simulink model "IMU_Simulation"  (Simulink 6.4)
settings: Solver=FixedStepDiscrete  StartTime=0.0  StopTime=25  FixedStep=.001  RelTol=1e-3
PreLoadFcn:
  | Script_Kalman
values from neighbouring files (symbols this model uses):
  Az = [1 -Ts ;0 1]    [Script_Kalman.m]
  Kz = 1e-3*[.4 ; -.04]    [Script_Kalman.m]
  Ts = .001    (= 0.001)    [Script_Kalman.m]
undefined symbols (not defined in the file or in its folder): dend, DiscIntNeverNeededParam, float, gaind, numd, polesd, tustin, zerosd
libraries: simulink x38
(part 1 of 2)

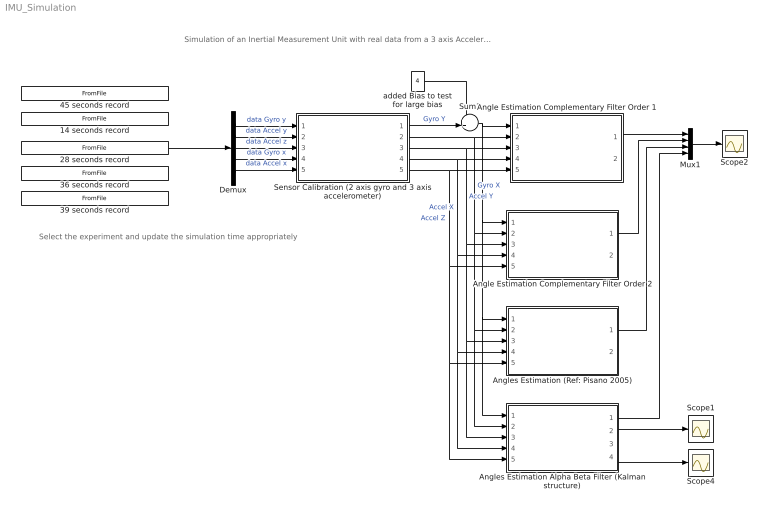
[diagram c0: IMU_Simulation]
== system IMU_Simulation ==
  note: Simulation of an Inertial Measurement Unit with real data from a 3 axis Accelerometer and 2 gyrometers Comparison between data fusion algorithms Find explanations at http://www.kerhuel.eu
  note: Select the experiment and update the simulation time appropriately
  14 seconds record : FromFile  FileName=Simulink_Static.mat  SampleTime=.001
  28 seconds record : FromFile  FileName=Simulink_Dynamic_Calibration2.mat  SampleTime=.001
  36 seconds record : FromFile  FileName=Simulink_Dynamic_Calibration.mat  SampleTime=.001
  39 seconds record : FromFile  FileName=Simulink_Dynamic_Calibration3.mat  SampleTime=.001
  45 seconds record : FromFile  FileName=Simulink_Static_60s.mat  SampleTime=.001
  Angle Estimation Complementary Filter Order 1 : Subsystem
  Angle Estimation Complementary Filter Order 2 : Subsystem
  Angles Estimation (Ref: Pisano 2005) : Subsystem
  Angles Estimation Alpha Beta Filter (Kalman structure) : Subsystem
  Demux : Demux  Outputs=5
  Mux1 : Mux
  Scope1 : Scope
  Scope2 : Scope
  Scope4 : Scope
  Sensor Calibration (2 axis gyro and 3 axis accelerometer) : Subsystem
  Sum1 : Sum  Inputs=++|  OutDataType=sfix(16)  OutScaling=2^0
  added Bias to test for large bias : Constant  Value=4  OutDataType=sfix(16)  OutScaling=2^0
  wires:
  Demux/2 -> Sensor Calibration (2 axis gyro and 3 axis accelerometer)/2(Accel Y)  "data Accel y"
  Demux/3 -> Sensor Calibration (2 axis gyro and 3 axis accelerometer)/3(Accel Z)  "data Accel z"
  Demux/4 -> Sensor Calibration (2 axis gyro and 3 axis accelerometer)/4(Gyro X)  "data Gyro x"
  Demux/5 -> Sensor Calibration (2 axis gyro and 3 axis accelerometer)/5(Accel X)  "data Accel x"
  Demux/1 -> Sensor Calibration (2 axis gyro and 3 axis accelerometer)/1(Gyro Y)  "data Gyro y"
  Sensor Calibration (2 axis gyro and 3 axis accelerometer)/1(Gyro Y (degree/s)) -> Sum1/2  "Gyro Y"
  Sensor Calibration (2 axis gyro and 3 axis accelerometer)/2(Gyro X (degree/s)) -> Angle Estimation Complementary Filter Order 1/2(Gyro X), Angles Estimation (Ref: Pisano 2005)/2(Gyro X), Angles Estimation Alpha Beta Filter (Kalman structure)/2(Gyro X), Angle Estimation Complementary Filter Order 2/2(Gyro X)  "Gyro X"
  Sensor Calibration (2 axis gyro and 3 axis accelerometer)/3(unbiased Accel Y) -> Angle Estimation Complementary Filter Order 1/3(Accel Y), Angles Estimation (Ref: Pisano 2005)/3(Accel Y), Angles Estimation Alpha Beta Filter (Kalman structure)/3(Accel Y), Angle Estimation Complementary Filter Order 2/3(Accel Y)  "Accel Y"
  Sensor Calibration (2 axis gyro and 3 axis accelerometer)/4(unbiased Accel X) -> Angle Estimation Complementary Filter Order 1/4(Accel X), Angles Estimation (Ref: Pisano 2005)/4(Accel X), Angles Estimation Alpha Beta Filter (Kalman structure)/4(Accel X), Angle Estimation Complementary Filter Order 2/4(Accel X)  "Accel X"
  Sensor Calibration (2 axis gyro and 3 axis accelerometer)/5(unbiased Accel Z) -> Angle Estimation Complementary Filter Order 1/5(Axxel Z (2)), Angles Estimation (Ref: Pisano 2005)/5(Accel Z), Angles Estimation Alpha Beta Filter (Kalman structure)/5(Accel Z), Angle Estimation Complementary Filter Order 2/5(Axxel Z (2))  "Accel Z"
  Mux1/1 -> Scope2/1
  Angle Estimation Complementary Filter Order 1/1(Angle Estimation Y) -> Mux1/1
  Angle Estimation Complementary Filter Order 2/1(Angle Estimation Y) -> Mux1/2
  Angles Estimation (Ref: Pisano 2005)/1(Angle Estimation Y) -> Mux1/3
  Angles Estimation Alpha Beta Filter (Kalman structure)/1(Angle Estimation Y) -> Mux1/4
  Sum1/1 -> Angle Estimation Complementary Filter Order 1/1("Gyro Y "), Angles Estimation (Ref: Pisano 2005)/1(Gyro Y), Angles Estimation Alpha Beta Filter (Kalman structure)/1(Gyro Y), Angle Estimation Complementary Filter Order 2/1("Gyro Y ")
  added Bias to test for large bias/1 -> Sum1/1
  Angles Estimation Alpha Beta Filter (Kalman structure)/2(Speed rate Axis Y1) -> Scope1/1
  Angles Estimation Alpha Beta Filter (Kalman structure)/4(Speed rate Axis X) -> Scope4/1
  28 seconds record/1 -> Demux/1

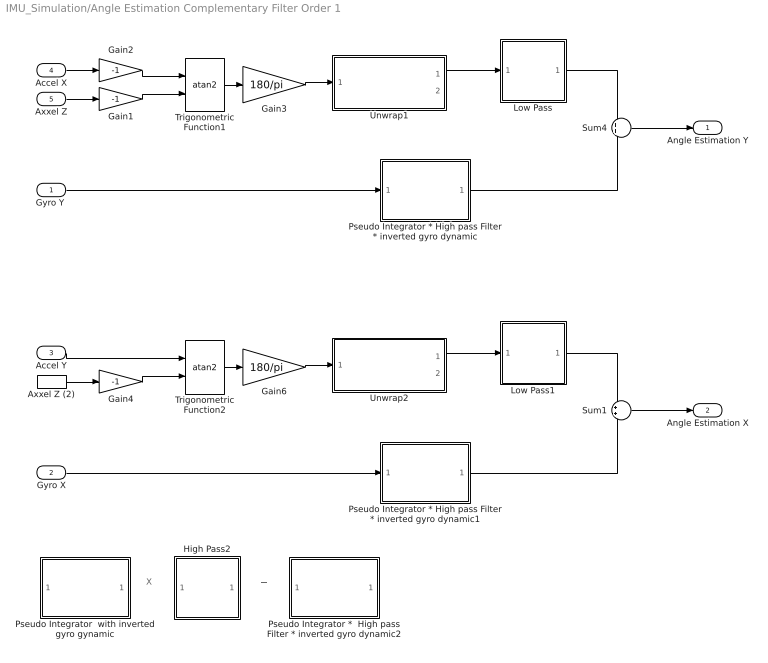
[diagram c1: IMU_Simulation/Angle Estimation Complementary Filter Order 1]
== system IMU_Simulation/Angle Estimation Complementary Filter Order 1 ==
  note: X
  note: =
  "Gyro Y " : Inport
  Gyro X : Inport  Port=2
  Accel Y : Inport  Port=3
  Accel X : Inport  Port=4
  Axxel Z : Inport  Port=5
  Axxel Z (2) : InportShadow  Port=5  LatchByCopyingInsideSignal=off
  Gain1 : Gain  Gain=-1  ParameterDataType=sfix(16)  ParameterScaling=2^0  OutDataType=sfix(16)  OutScaling=2^0
  Gain2 : Gain  Gain=-1  ParameterDataType=sfix(16)  ParameterScaling=2^0  OutDataType=sfix(16)  OutScaling=2^0
  Gain3 : Gain  Gain=180/pi  ParameterDataType=sfix(16)  ParameterScaling=2^0  OutDataTypeMode=Specify via dialog  OutDataType=float('double')
  Gain4 : Gain  Gain=-1  ParameterDataType=sfix(16)  ParameterScaling=2^0  OutDataType=sfix(16)  OutScaling=2^0
  Gain6 : Gain  Gain=180/pi  ParameterDataType=sfix(16)  ParameterScaling=2^0  OutDataTypeMode=Specify via dialog  OutDataType=float('double')
  High Pass2 : Subsystem  mask(DiscretizedZeroPole){Zeros=[0], Poles=[-.5], Gain=1, AbsTol=auto, SampleTime=.001, method=tustin, Wc=1}
      mask prompts: Zeros "Zeros (enter in s-main:)"; Poles "Poles (enter in s-domain:)"; Gain "Gain (enter in s-domain:)"; AbsTol "Absolute tolerance:"; SampleTime "Sample time:"; Wc "Critical Frequency (Hz):"
      mask help: Continuous mask uses c2d to transform parameters onto the Discrete Zero-Pole block inside.
      mask init:
      | st=SampleTime;
      | if length(st)>1
      |     st=SampleTime(1);
      | end
      | if(st>0)
      |     [zerosd,polesd,gaind] = sldiscutil('disczpk', {st,method,Wc,Zeros,Poles,Gain});
      | end	
      | s = get_param(gcb,'maskvalues');
      | zeross = s{1};
      | poless = s{2};
      | gainss = s{3};
      | %zerosc = eval(zeross);
      | %polesc = eval(poless);
      | %gainsc = eval(gainss);
      | sldiscutil('initzpkmask', st);
      | if(st==0)
      | set_param([gcb '/Zero Pole'], 'AbsoluteTolerance', AbsTol);
      | end
  Low Pass : Subsystem  mask(DiscretizedZeroPole){Zeros=[], Poles=[-.5], Gain=.5, AbsTol=auto, SampleTime=.001, method=tustin, Wc=1}
      mask prompts: Zeros "Zeros (enter in s-main:)"; Poles "Poles (enter in s-domain:)"; Gain "Gain (enter in s-domain:)"; AbsTol "Absolute tolerance:"; SampleTime "Sample time:"; Wc "Critical Frequency (Hz):"
      mask help: Continuous mask uses c2d to transform parameters onto the Discrete Zero-Pole block inside.
      mask init:
      | st=SampleTime;
      | if length(st)>1
      |     st=SampleTime(1);
      | end
      | if(st>0)
      |     [zerosd,polesd,gaind] = sldiscutil('disczpk', {st,method,Wc,Zeros,Poles,Gain});
      | end	
      | s = get_param(gcb,'maskvalues');
      | zeross = s{1};
      | poless = s{2};
      | gainss = s{3};
      | %zerosc = eval(zeross);
      | %polesc = eval(poless);
      | %gainsc = eval(gainss);
      | sldiscutil('initzpkmask', st);
      | if(st==0)
      | set_param([gcb '/Zero Pole'], 'AbsoluteTolerance', AbsTol);
      | end
  Low Pass1 : Subsystem  mask(DiscretizedZeroPole){Zeros=[], Poles=[-.5], Gain=.5, AbsTol=auto, SampleTime=.001, method=tustin, Wc=1}
      mask prompts: Zeros "Zeros (enter in s-main:)"; Poles "Poles (enter in s-domain:)"; Gain "Gain (enter in s-domain:)"; AbsTol "Absolute tolerance:"; SampleTime "Sample time:"; Wc "Critical Frequency (Hz):"
      mask help: Continuous mask uses c2d to transform parameters onto the Discrete Zero-Pole block inside.
      mask init:
      | st=SampleTime;
      | if length(st)>1
      |     st=SampleTime(1);
      | end
      | if(st>0)
      |     [zerosd,polesd,gaind] = sldiscutil('disczpk', {st,method,Wc,Zeros,Poles,Gain});
      | end	
      | s = get_param(gcb,'maskvalues');
      | zeross = s{1};
      | poless = s{2};
      | gainss = s{3};
      | %zerosc = eval(zeross);
      | %polesc = eval(poless);
      | %gainsc = eval(gainss);
      | sldiscutil('initzpkmask', st);
      | if(st==0)
      | set_param([gcb '/Zero Pole'], 'AbsoluteTolerance', AbsTol);
      | end
  Pseudo Integrator  with inverted gyro gynamic : Subsystem  mask(DiscretizedZeroPole){Zeros=[-314], Poles=[0], Gain=(1/314), AbsTol=auto, SampleTime=.001, method=tustin, Wc=1}
      mask prompts: Zeros "Zeros (enter in s-main:)"; Poles "Poles (enter in s-domain:)"; Gain "Gain (enter in s-domain:)"; AbsTol "Absolute tolerance:"; SampleTime "Sample time:"; Wc "Critical Frequency (Hz):"
      mask help: Continuous mask uses c2d to transform parameters onto the Discrete Zero-Pole block inside.
      mask init:
      | st=SampleTime;
      | if length(st)>1
      |     st=SampleTime(1);
      | end
      | if(st>0)
      |     [zerosd,polesd,gaind] = sldiscutil('disczpk', {st,method,Wc,Zeros,Poles,Gain});
      | end	
      | s = get_param(gcb,'maskvalues');
      | zeross = s{1};
      | poless = s{2};
      | gainss = s{3};
      | %zerosc = eval(zeross);
      | %polesc = eval(poless);
      | %gainsc = eval(gainss);
      | sldiscutil('initzpkmask', st);
      | if(st==0)
      | set_param([gcb '/Zero Pole'], 'AbsoluteTolerance', AbsTol);
      | end
  Pseudo Integrator *  High pass Filter * inverted gyro dynamic2 : Subsystem  mask(DiscretizedZeroPole){Zeros=[-314], Poles=[-.5], Gain=(1/314), AbsTol=auto, SampleTime=.001, method=tustin, Wc=1}
      mask prompts: Zeros "Zeros (enter in s-main:)"; Poles "Poles (enter in s-domain:)"; Gain "Gain (enter in s-domain:)"; AbsTol "Absolute tolerance:"; SampleTime "Sample time:"; Wc "Critical Frequency (Hz):"
      mask help: Continuous mask uses c2d to transform parameters onto the Discrete Zero-Pole block inside.
      mask init:
      | st=SampleTime;
      | if length(st)>1
      |     st=SampleTime(1);
      | end
      | if(st>0)
      |     [zerosd,polesd,gaind] = sldiscutil('disczpk', {st,method,Wc,Zeros,Poles,Gain});
      | end	
      | s = get_param(gcb,'maskvalues');
      | zeross = s{1};
      | poless = s{2};
      | gainss = s{3};
      | %zerosc = eval(zeross);
      | %polesc = eval(poless);
      | %gainsc = eval(gainss);
      | sldiscutil('initzpkmask', st);
      | if(st==0)
      | set_param([gcb '/Zero Pole'], 'AbsoluteTolerance', AbsTol);
      | end
  Pseudo Integrator * High pass Filter * inverted gyro dynamic : Subsystem  mask(DiscretizedZeroPole){Zeros=[-314], Poles=[-.5], Gain=(1/314), AbsTol=auto, SampleTime=.001, method=tustin, Wc=1}
      mask prompts: Zeros "Zeros (enter in s-main:)"; Poles "Poles (enter in s-domain:)"; Gain "Gain (enter in s-domain:)"; AbsTol "Absolute tolerance:"; SampleTime "Sample time:"; Wc "Critical Frequency (Hz):"
      mask help: Continuous mask uses c2d to transform parameters onto the Discrete Zero-Pole block inside.
      mask init:
      | st=SampleTime;
      | if length(st)>1
      |     st=SampleTime(1);
      | end
      | if(st>0)
      |     [zerosd,polesd,gaind] = sldiscutil('disczpk', {st,method,Wc,Zeros,Poles,Gain});
      | end	
      | s = get_param(gcb,'maskvalues');
      | zeross = s{1};
      | poless = s{2};
      | gainss = s{3};
      | %zerosc = eval(zeross);
      | %polesc = eval(poless);
      | %gainsc = eval(gainss);
      | sldiscutil('initzpkmask', st);
      | if(st==0)
      | set_param([gcb '/Zero Pole'], 'AbsoluteTolerance', AbsTol);
      | end
  Pseudo Integrator * High pass Filter * inverted gyro dynamic1 : Subsystem  mask(DiscretizedZeroPole){Zeros=[-314], Poles=[-.5], Gain=(1/314), AbsTol=auto, SampleTime=.001, method=tustin, Wc=1}
      mask prompts: Zeros "Zeros (enter in s-main:)"; Poles "Poles (enter in s-domain:)"; Gain "Gain (enter in s-domain:)"; AbsTol "Absolute tolerance:"; SampleTime "Sample time:"; Wc "Critical Frequency (Hz):"
      mask help: Continuous mask uses c2d to transform parameters onto the Discrete Zero-Pole block inside.
      mask init:
      | st=SampleTime;
      | if length(st)>1
      |     st=SampleTime(1);
      | end
      | if(st>0)
      |     [zerosd,polesd,gaind] = sldiscutil('disczpk', {st,method,Wc,Zeros,Poles,Gain});
      | end	
      | s = get_param(gcb,'maskvalues');
      | zeross = s{1};
      | poless = s{2};
      | gainss = s{3};
      | %zerosc = eval(zeross);
      | %polesc = eval(poless);
      | %gainsc = eval(gainss);
      | sldiscutil('initzpkmask', st);
      | if(st==0)
      | set_param([gcb '/Zero Pole'], 'AbsoluteTolerance', AbsTol);
      | end
  Sum1 : Sum  OutDataType=sfix(16)  OutScaling=2^0
  Sum4 : Sum  OutDataType=sfix(16)  OutScaling=2^0
  Trigonometric Function1 : Trigonometry  Operator=atan2  OutputSignalType=real
  Trigonometric Function2 : Trigonometry  Operator=atan2  OutputSignalType=real
  Unwrap1 : Subsystem
  Unwrap2 : Subsystem
  Angle Estimation Y : Outport
  Angle Estimation X : Outport  Port=2
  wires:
  Unwrap2/1(unwrap angle) -> Low Pass1/1(In1)
  Gain6/1 -> Unwrap2/1(Estimated Angle)
  Trigonometric Function2/1 -> Gain6/1
  Gain4/1 -> Trigonometric Function2/2
  Gyro X/1 -> Pseudo Integrator * High pass Filter * inverted gyro dynamic1/1(In1)
  Sum1/1 -> Angle Estimation X/1
  Axxel Z (2)/1 -> Gain4/1
  Accel Y/1 -> Trigonometric Function2/1
  Low Pass1/1(Out1) -> Sum1/1
  Unwrap1/1(unwrap angle) -> Low Pass/1(In1)
  Gain3/1 -> Unwrap1/1(Estimated Angle)
  Trigonometric Function1/1 -> Gain3/1
  Gain1/1 -> Trigonometric Function1/2
  Gain2/1 -> Trigonometric Function1/1
  "Gyro Y "/1 -> Pseudo Integrator * High pass Filter * inverted gyro dynamic/1(In1)
  Sum4/1 -> Angle Estimation Y/1
  Axxel Z/1 -> Gain1/1
  Accel X/1 -> Gain2/1
  Low Pass/1(Out1) -> Sum4/1
  Pseudo Integrator * High pass Filter * inverted gyro dynamic1/1(Out1) -> Sum1/2
  Pseudo Integrator * High pass Filter * inverted gyro dynamic/1(Out1) -> Sum4/2

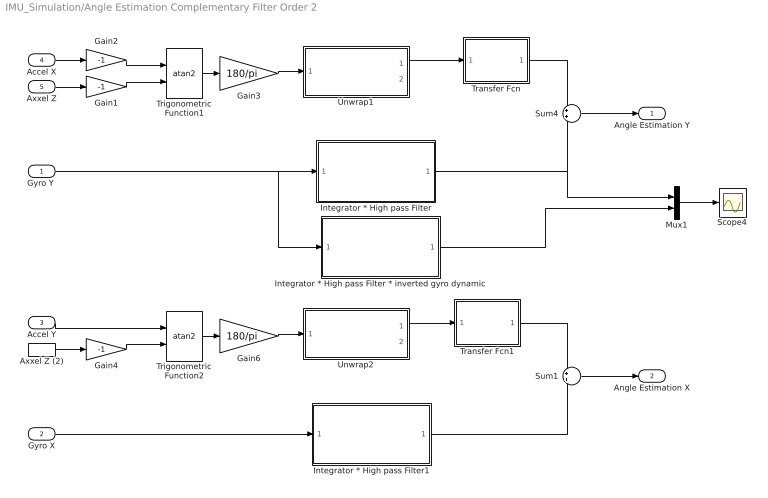
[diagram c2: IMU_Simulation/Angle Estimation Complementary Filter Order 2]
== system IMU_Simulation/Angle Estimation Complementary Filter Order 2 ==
  "Gyro Y " : Inport
  Gyro X : Inport  Port=2
  Accel Y : Inport  Port=3
  Accel X : Inport  Port=4
  Axxel Z : Inport  Port=5
  Axxel Z (2) : InportShadow  Port=5  LatchByCopyingInsideSignal=off
  Gain1 : Gain  Gain=-1  ParameterDataType=sfix(16)  ParameterScaling=2^0  OutDataType=sfix(16)  OutScaling=2^0
  Gain2 : Gain  Gain=-1  ParameterDataType=sfix(16)  ParameterScaling=2^0  OutDataType=sfix(16)  OutScaling=2^0
  Gain3 : Gain  Gain=180/pi  ParameterDataType=sfix(16)  ParameterScaling=2^0  OutDataTypeMode=Specify via dialog  OutDataType=float('double')
  Gain4 : Gain  Gain=-1  ParameterDataType=sfix(16)  ParameterScaling=2^0  OutDataType=sfix(16)  OutScaling=2^0
  Gain6 : Gain  Gain=180/pi  ParameterDataType=sfix(16)  ParameterScaling=2^0  OutDataTypeMode=Specify via dialog  OutDataType=float('double')
  Integrator * High pass Filter : Subsystem  mask(DiscretizedZeroPole){Zeros=[0], Poles=[-.2 -.2], Gain=1, AbsTol=auto, SampleTime=.001, method=tustin, Wc=1}
      mask prompts: Zeros "Zeros (enter in s-main:)"; Poles "Poles (enter in s-domain:)"; Gain "Gain (enter in s-domain:)"; AbsTol "Absolute tolerance:"; SampleTime "Sample time:"; Wc "Critical Frequency (Hz):"
      mask help: Continuous mask uses c2d to transform parameters onto the Discrete Zero-Pole block inside.
      mask init:
      | st=SampleTime;
      | if length(st)>1
      |     st=SampleTime(1);
      | end
      | if(st>0)
      |     [zerosd,polesd,gaind] = sldiscutil('disczpk', {st,method,Wc,Zeros,Poles,Gain});
      | end	
      | s = get_param(gcb,'maskvalues');
      | zeross = s{1};
      | poless = s{2};
      | gainss = s{3};
      | %zerosc = eval(zeross);
      | %polesc = eval(poless);
      | %gainsc = eval(gainss);
      | sldiscutil('initzpkmask', st);
      | if(st==0)
      | set_param([gcb '/Zero Pole'], 'AbsoluteTolerance', AbsTol);
      | end
  Integrator * High pass Filter * inverted gyro dynamic : Subsystem  mask(DiscretizedZeroPole){Zeros=[-314 0], Poles=[-.2 -.2], Gain=(1/314), AbsTol=auto, SampleTime=.001, method=tustin, Wc=1}
      mask prompts: Zeros "Zeros (enter in s-main:)"; Poles "Poles (enter in s-domain:)"; Gain "Gain (enter in s-domain:)"; AbsTol "Absolute tolerance:"; SampleTime "Sample time:"; Wc "Critical Frequency (Hz):"
      mask help: Continuous mask uses c2d to transform parameters onto the Discrete Zero-Pole block inside.
      mask init:
      | st=SampleTime;
      | if length(st)>1
      |     st=SampleTime(1);
      | end
      | if(st>0)
      |     [zerosd,polesd,gaind] = sldiscutil('disczpk', {st,method,Wc,Zeros,Poles,Gain});
      | end	
      | s = get_param(gcb,'maskvalues');
      | zeross = s{1};
      | poless = s{2};
      | gainss = s{3};
      | %zerosc = eval(zeross);
      | %polesc = eval(poless);
      | %gainsc = eval(gainss);
      | sldiscutil('initzpkmask', st);
      | if(st==0)
      | set_param([gcb '/Zero Pole'], 'AbsoluteTolerance', AbsTol);
      | end
  Integrator * High pass Filter1 : Subsystem  mask(DiscretizedZeroPole){Zeros=[0], Poles=[-.2 -.2], Gain=1, AbsTol=auto, SampleTime=.001, method=tustin, Wc=1}
      mask prompts: Zeros "Zeros (enter in s-main:)"; Poles "Poles (enter in s-domain:)"; Gain "Gain (enter in s-domain:)"; AbsTol "Absolute tolerance:"; SampleTime "Sample time:"; Wc "Critical Frequency (Hz):"
      mask help: Continuous mask uses c2d to transform parameters onto the Discrete Zero-Pole block inside.
      mask init:
      | st=SampleTime;
      | if length(st)>1
      |     st=SampleTime(1);
      | end
      | if(st>0)
      |     [zerosd,polesd,gaind] = sldiscutil('disczpk', {st,method,Wc,Zeros,Poles,Gain});
      | end	
      | s = get_param(gcb,'maskvalues');
      | zeross = s{1};
      | poless = s{2};
      | gainss = s{3};
      | %zerosc = eval(zeross);
      | %polesc = eval(poless);
      | %gainsc = eval(gainss);
      | sldiscutil('initzpkmask', st);
      | if(st==0)
      | set_param([gcb '/Zero Pole'], 'AbsoluteTolerance', AbsTol);
      | end
  Mux1 : Mux  Inputs=2
  Scope4 : Scope
  Sum1 : Sum  OutDataType=sfix(16)  OutScaling=2^0
  Sum4 : Sum  OutDataType=sfix(16)  OutScaling=2^0
  Transfer Fcn : Subsystem  mask(DiscretizedTransferFcn){Numerator=[.4 .02], Denominator=[1 .4 .02], AbsTol=auto, SampleTime=.001, method=tustin, Wc=0}
      mask prompts: Numerator "Numerator (enter in s-domain:)"; Denominator "Denominator (enter in s-domain:)"; AbsTol "Absolute tolerance:"; SampleTime "Sample time:"; Wc "Critical Frequency (Hz):"
      mask help: Continuous mask uses c2d to transform parameters onto the Discrete Transfer function block inside.
      mask init:
      | st=SampleTime;
      | if length(st)>1
      |     st=SampleTime(1);
      | end
      | if(st>0)
      |     [numd,dend] = sldiscutil('disctransferfcn',{st,method,Wc,Numerator,Denominator});
      | end	
      | s = get_param(gcb,'maskvalues');
      | nums = s{1};
      | dens = s{2};
      | %numc = eval(nums);
      | %denc = eval(dens);
      | sldiscutil('inittfmask', st);
      | if(st==0)
      | set_param([gcb '/Transfer Fcn'], 'AbsoluteTolerance', AbsTol);
      | end
  Transfer Fcn1 : Subsystem  mask(DiscretizedTransferFcn){Numerator=[.4 .02], Denominator=[1 .4 .02], AbsTol=auto, SampleTime=.001, method=tustin, Wc=0}
      mask prompts: Numerator "Numerator (enter in s-domain:)"; Denominator "Denominator (enter in s-domain:)"; AbsTol "Absolute tolerance:"; SampleTime "Sample time:"; Wc "Critical Frequency (Hz):"
      mask help: Continuous mask uses c2d to transform parameters onto the Discrete Transfer function block inside.
      mask init:
      | st=SampleTime;
      | if length(st)>1
      |     st=SampleTime(1);
      | end
      | if(st>0)
      |     [numd,dend] = sldiscutil('disctransferfcn',{st,method,Wc,Numerator,Denominator});
      | end	
      | s = get_param(gcb,'maskvalues');
      | nums = s{1};
      | dens = s{2};
      | %numc = eval(nums);
      | %denc = eval(dens);
      | sldiscutil('inittfmask', st);
      | if(st==0)
      | set_param([gcb '/Transfer Fcn'], 'AbsoluteTolerance', AbsTol);
      | end
  Trigonometric Function1 : Trigonometry  Operator=atan2  OutputSignalType=real
  Trigonometric Function2 : Trigonometry  Operator=atan2  OutputSignalType=real
  Unwrap1 : Subsystem
  Unwrap2 : Subsystem
  Angle Estimation Y : Outport
  Angle Estimation X : Outport  Port=2
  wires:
  Integrator * High pass Filter/1(Out1) -> Sum4/2, Mux1/1
  Integrator * High pass Filter1/1(Out1) -> Sum1/2
  Transfer Fcn/1(Out1) -> Sum4/1
  Accel X/1 -> Gain2/1
  Axxel Z/1 -> Gain1/1
  Sum4/1 -> Angle Estimation Y/1
  "Gyro Y "/1 -> Integrator * High pass Filter/1(In1), Integrator * High pass Filter * inverted gyro dynamic/1(In1)
  Gain2/1 -> Trigonometric Function1/1
  Gain1/1 -> Trigonometric Function1/2
  Trigonometric Function1/1 -> Gain3/1
  Gain3/1 -> Unwrap1/1(Estimated Angle)
  Unwrap1/1(unwrap angle) -> Transfer Fcn/1(In1)
  Transfer Fcn1/1(Out1) -> Sum1/1
  Accel Y/1 -> Trigonometric Function2/1
  Axxel Z (2)/1 -> Gain4/1
  Sum1/1 -> Angle Estimation X/1
  Gyro X/1 -> Integrator * High pass Filter1/1(In1)
  Gain4/1 -> Trigonometric Function2/2
  Trigonometric Function2/1 -> Gain6/1
  Gain6/1 -> Unwrap2/1(Estimated Angle)
  Unwrap2/1(unwrap angle) -> Transfer Fcn1/1(In1)
  Integrator * High pass Filter * inverted gyro dynamic/1(Out1) -> Mux1/2
  Mux1/1 -> Scope4/1

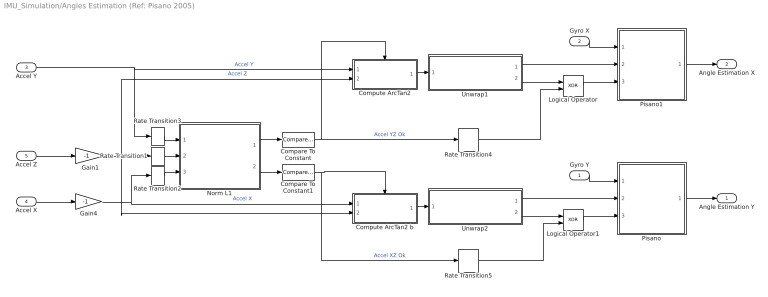
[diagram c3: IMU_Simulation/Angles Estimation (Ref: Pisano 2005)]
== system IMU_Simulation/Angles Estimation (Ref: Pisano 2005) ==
  Gyro Y : Inport
  Gyro X : Inport  Port=2
  Accel Y : Inport  Port=3
  Accel X : Inport  Port=4
  Accel Z : Inport  Port=5
  Compare To Constant : simulink/Logic and Bit Operations/Compare To Constant  SystemSampleTime=-1  relop=>=  const=200  LogicOutDataTypeMode=boolean  ZeroCross=off
  Compare To Constant1 : simulink/Logic and Bit Operations/Compare To Constant  SystemSampleTime=-1  relop=>=  const=200  LogicOutDataTypeMode=boolean  ZeroCross=off
  Compute ArcTan2 : Subsystem
  Compute ArcTan2 b : Subsystem
  Gain1 : Gain  Gain=-1  ParameterDataType=sfix(16)  ParameterScaling=2^0  OutDataType=sfix(16)  OutScaling=2^0
  Gain4 : Gain  Gain=-1  ParameterDataType=sfix(16)  ParameterScaling=2^0  OutDataType=sfix(16)  OutScaling=2^0
  Logical Operator : Logic  Operator=XOR  AllPortsSameDT=off  OutDataTypeMode=boolean
  Logical Operator1 : Logic  Operator=XOR  AllPortsSameDT=off  OutDataTypeMode=boolean
  Norm L1 : Subsystem
  Pisano : Subsystem
  Pisano1 : Subsystem
  Rate Transition1 : RateTransition  Integrity=off  OutPortSampleTime=.2
  Rate Transition2 : RateTransition  Integrity=off  OutPortSampleTime=.2
  Rate Transition3 : RateTransition  Integrity=off  OutPortSampleTime=.2
  Rate Transition4 : RateTransition  Integrity=off  OutPortSampleTime=.001
  Rate Transition5 : RateTransition  Integrity=off  OutPortSampleTime=.001
  Unwrap1 : Subsystem
  Unwrap2 : Subsystem
  Angle Estimation Y : Outport
  Angle Estimation X : Outport  Port=2
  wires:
  Pisano/1(Position) -> Angle Estimation Y/1
  Unwrap2/1(unwrap angle) -> Pisano/2(Accel)
  Unwrap2/2(Wrap) -> Logical Operator1/1
  Logical Operator/1 -> Pisano1/3(Adapt)
  Rate Transition5/1 -> Logical Operator1/2
  Gain1/1 -> Rate Transition1/1, Compute ArcTan2/2(Force 2), Compute ArcTan2 b/2(Force 2)  "Accel Z"
  Logical Operator1/1 -> Pisano/3(Adapt)
  Rate Transition4/1 -> Logical Operator/2
  Unwrap1/2(Wrap) -> Logical Operator/1
  Unwrap1/1(unwrap angle) -> Pisano1/2(Accel)
  Rate Transition3/1 -> Norm L1/1(Accel Y)
  Rate Transition2/1 -> Norm L1/3(Accel X)
  Rate Transition1/1 -> Norm L1/2(Accel Z)
  Compare To Constant1/1 -> Rate Transition5/1, Compute ArcTan2 b/Enable  "Accel XZ Ok"
  Compare To Constant/1 -> Rate Transition4/1, Compute ArcTan2/Enable  "Accel YZ Ok"
  Norm L1/1(abs(Y)+abs(Z)) -> Compare To Constant/1
  Norm L1/2(abs(X)+abs(Z)) -> Compare To Constant1/1
  Accel Z/1 -> Gain1/1
  Gain4/1 -> Rate Transition2/1, Compute ArcTan2 b/1(Force 1)  "Accel X"
  Compute ArcTan2/1(Degree) -> Unwrap1/1(Estimated Angle)
  Compute ArcTan2 b/1(Degree) -> Unwrap2/1(Estimated Angle)
  Accel X/1 -> Gain4/1
  Accel Y/1 -> Compute ArcTan2/1(Force 1), Rate Transition3/1  "Accel Y"
  Gyro X/1 -> Pisano1/1(Gyro)
  Gyro Y/1 -> Pisano/1(Gyro)
  Pisano1/1(Position) -> Angle Estimation X/1

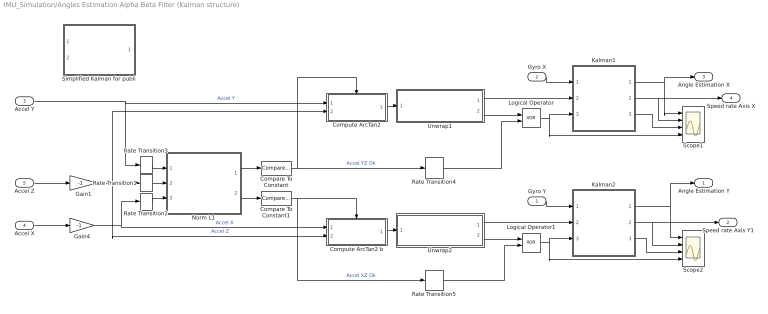
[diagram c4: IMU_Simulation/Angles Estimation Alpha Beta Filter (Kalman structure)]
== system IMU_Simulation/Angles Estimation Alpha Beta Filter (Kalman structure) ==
  Gyro Y : Inport
  Gyro X : Inport  Port=2
  Accel Y : Inport  Port=3
  Accel X : Inport  Port=4
  Accel Z : Inport  Port=5
  Compare To Constant : simulink/Logic and Bit Operations/Compare To Constant  SystemSampleTime=-1  relop=>=  const=200  LogicOutDataTypeMode=boolean  ZeroCross=off
  Compare To Constant1 : simulink/Logic and Bit Operations/Compare To Constant  SystemSampleTime=-1  relop=>=  const=200  LogicOutDataTypeMode=boolean  ZeroCross=off
  Compute ArcTan2 : Subsystem
  Compute ArcTan2 b : Subsystem
  Gain1 : Gain  Gain=-1  ParameterDataType=sfix(16)  ParameterScaling=2^0  OutDataType=sfix(16)  OutScaling=2^0
  Gain4 : Gain  Gain=-1  ParameterDataType=sfix(16)  ParameterScaling=2^0  OutDataType=sfix(16)  OutScaling=2^0
  Kalman1 : Subsystem
  Kalman2 : Subsystem
  Logical Operator : Logic  Operator=XOR  AllPortsSameDT=off  OutDataTypeMode=boolean
  Logical Operator1 : Logic  Operator=XOR  AllPortsSameDT=off  OutDataTypeMode=boolean
  Norm L1 : Subsystem
  Rate Transition1 : RateTransition  Integrity=off  OutPortSampleTime=.2
  Rate Transition2 : RateTransition  Integrity=off  OutPortSampleTime=.2
  Rate Transition3 : RateTransition  Integrity=off  OutPortSampleTime=.2
  Rate Transition4 : RateTransition  Integrity=off  OutPortSampleTime=.001
  Rate Transition5 : RateTransition  Integrity=off  OutPortSampleTime=.001
  Scope1 : Scope  NumInputPorts=4
  Scope2 : Scope  NumInputPorts=4
  Simplified Kalman for publi : Subsystem
  Unwrap1 : Subsystem
  Unwrap2 : Subsystem
  Angle Estimation Y : Outport
  Speed rate Axis Y1 : Outport  Port=2
  Angle Estimation X : Outport  Port=3
  Speed rate Axis X : Outport  Port=4
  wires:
  Gyro Y/1 -> Kalman2/1(Gyro)
  Gyro X/1 -> Kalman1/1(Gyro)
  Accel Y/1 -> Rate Transition3/1, Compute ArcTan2/1(Force 1)  "Accel Y"
  Accel X/1 -> Gain4/1
  Compute ArcTan2 b/1(Degree) -> Unwrap2/1(Estimated Angle)
  Compute ArcTan2/1(Degree) -> Unwrap1/1(Estimated Angle)
  Gain4/1 -> Compute ArcTan2 b/1(Force 1), Rate Transition2/1  "Accel X"
  Accel Z/1 -> Gain1/1
  Norm L1/2(abs(X)+abs(Z)) -> Compare To Constant1/1
  Norm L1/1(abs(Y)+abs(Z)) -> Compare To Constant/1
  Compare To Constant/1 -> Compute ArcTan2/Enable, Rate Transition4/1  "Accel YZ Ok"
  Compare To Constant1/1 -> Compute ArcTan2 b/Enable, Rate Transition5/1  "Accel XZ Ok"
  Kalman1/1(Position) -> Angle Estimation X/1, Scope1/1
  Kalman2/1(Position) -> Angle Estimation Y/1, Scope2/1
  Rate Transition1/1 -> Norm L1/2(Accel Z)
  Rate Transition2/1 -> Norm L1/3(Accel X)
  Rate Transition3/1 -> Norm L1/1(Accel Y)
  Unwrap1/1(unwrap angle) -> Kalman1/2(Accel1)
  Unwrap1/2(Wrap) -> Logical Operator/1
  Rate Transition4/1 -> Logical Operator/2
  Logical Operator1/1 -> Scope2/4, Kalman2/3(Adapt1)
  Gain1/1 -> Compute ArcTan2 b/2(Force 2), Compute ArcTan2/2(Force 2), Rate Transition1/1  "Accel Z"
  Rate Transition5/1 -> Logical Operator1/2
  Logical Operator/1 -> Kalman1/3(Adapt1), Scope1/4
  Unwrap2/2(Wrap) -> Logical Operator1/1
  Unwrap2/1(unwrap angle) -> Kalman2/2(Accel1)
  Kalman1/2(Speed) -> Scope1/2, Speed rate Axis X/1
  Kalman2/2(Speed) -> Scope2/2, Speed rate Axis Y1/1
  Kalman2/3(Bias) -> Scope2/3
  Kalman1/3(Bias) -> Scope1/3

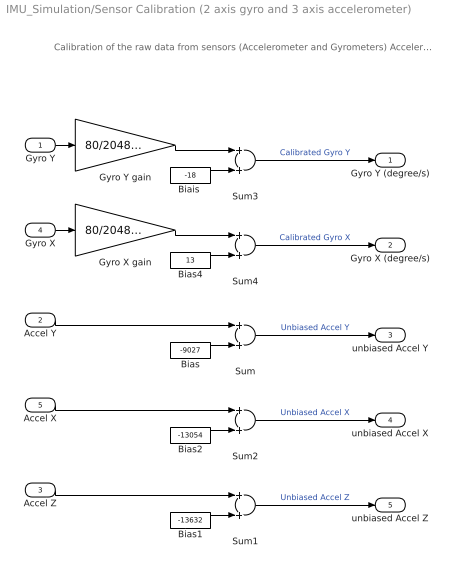
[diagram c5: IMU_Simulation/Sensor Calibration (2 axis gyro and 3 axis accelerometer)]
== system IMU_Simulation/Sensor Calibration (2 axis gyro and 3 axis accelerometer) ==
  note: Calibration of the raw data from sensors (Accelerometer and Gyrometers) Accelerometer do not need any gain because the Arctan function used compute a raport of two acceleration Gyro needs gain and bias calibration. From the sensor doc, the gain should be 80/2048 but...
  Gyro Y : Inport
  Accel Y : Inport  Port=2
  Accel Z : Inport  Port=3
  Gyro X : Inport  Port=4
  Accel X : Inport  Port=5
  "Biais " : Constant  Value=-18  OutDataType=sfix(16)  OutScaling=2^0
  Bias : Constant  Value=-9027  OutDataType=sfix(16)  OutScaling=2^0
  Bias1 : Constant  Value=-13632  OutDataType=sfix(16)  OutScaling=2^0
  Bias2 : Constant  Value=-13054  OutDataType=sfix(16)  OutScaling=2^0
  Bias4 : Constant  Value=13  OutDataType=sfix(16)  OutScaling=2^0
  Gyro X gain : Gain  Gain=80/2048*2.35  ParameterDataType=sfix(16)  ParameterScaling=2^0  OutDataTypeMode=Specify via dialog  OutDataType=float('double')
  Gyro Y gain : Gain  Gain=80/2048*6.55  ParameterDataType=sfix(16)  ParameterScaling=2^0  OutDataTypeMode=Specify via dialog  OutDataType=float('double')
  Sum{,1..4} (5 alike) : Sum  OutDataType=sfix(16)  OutScaling=2^0
  Gyro Y (degree/s) : Outport
  Gyro X (degree/s) : Outport  Port=2
  unbiased Accel Y : Outport  Port=3
  unbiased Accel X : Outport  Port=4
  unbiased Accel Z : Outport  Port=5
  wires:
  Bias/1 -> Sum/2
  Bias1/1 -> Sum1/2
  Bias2/1 -> Sum2/2
  Gyro Y/1 -> Gyro Y gain/1
  Accel Y/1 -> Sum/1
  Sum/1 -> unbiased Accel Y/1  "Unbiased Accel Y"
  Accel Z/1 -> Sum1/1
  Sum1/1 -> unbiased Accel Z/1  "Unbiased Accel Z"
  Gyro X/1 -> Gyro X gain/1
  Accel X/1 -> Sum2/1
  Sum2/1 -> unbiased Accel X/1  "Unbiased Accel X"
  Gyro Y gain/1 -> Sum3/1
  Sum3/1 -> Gyro Y (degree/s)/1  "Calibrated Gyro Y"
  "Biais "/1 -> Sum3/2
  Gyro X gain/1 -> Sum4/1
  Sum4/1 -> Gyro X (degree/s)/1  "Calibrated Gyro X"
  Bias4/1 -> Sum4/2

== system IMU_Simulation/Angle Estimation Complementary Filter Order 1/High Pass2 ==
  In1 : Inport  OutDataType=sfix(16)  OutScaling=2^0
  Discrete Zero-Pole : DiscreteZeroPole  Zeros=zerosd  Poles=polesd  Gain=gaind  SampleTime=SampleTime
  Out1 : Outport  OutDataType=sfix(16)  OutScaling=2^0
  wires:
  Discrete Zero-Pole/1 -> Out1/1
  In1/1 -> Discrete Zero-Pole/1

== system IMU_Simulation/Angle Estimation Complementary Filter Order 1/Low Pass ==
  In1 : Inport  OutDataType=sfix(16)  OutScaling=2^0
  Discrete Zero-Pole : DiscreteZeroPole  Zeros=zerosd  Poles=polesd  Gain=gaind  SampleTime=SampleTime
  Out1 : Outport  OutDataType=sfix(16)  OutScaling=2^0
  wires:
  Discrete Zero-Pole/1 -> Out1/1
  In1/1 -> Discrete Zero-Pole/1

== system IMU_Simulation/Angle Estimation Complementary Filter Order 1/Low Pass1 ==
  In1 : Inport  OutDataType=sfix(16)  OutScaling=2^0
  Discrete Zero-Pole : DiscreteZeroPole  Zeros=zerosd  Poles=polesd  Gain=gaind  SampleTime=SampleTime
  Out1 : Outport  OutDataType=sfix(16)  OutScaling=2^0
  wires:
  In1/1 -> Discrete Zero-Pole/1
  Discrete Zero-Pole/1 -> Out1/1

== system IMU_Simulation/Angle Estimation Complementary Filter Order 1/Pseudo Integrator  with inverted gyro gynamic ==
  In1 : Inport  OutDataType=sfix(16)  OutScaling=2^0
  Discrete Zero-Pole : DiscreteZeroPole  Zeros=zerosd  Poles=polesd  Gain=gaind  SampleTime=SampleTime
  Out1 : Outport  OutDataType=sfix(16)  OutScaling=2^0
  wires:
  Discrete Zero-Pole/1 -> Out1/1
  In1/1 -> Discrete Zero-Pole/1

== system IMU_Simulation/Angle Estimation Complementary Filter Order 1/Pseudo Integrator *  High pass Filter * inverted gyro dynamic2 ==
  In1 : Inport  OutDataType=sfix(16)  OutScaling=2^0
  Discrete Zero-Pole : DiscreteZeroPole  Zeros=zerosd  Poles=polesd  Gain=gaind  SampleTime=SampleTime
  Out1 : Outport  OutDataType=sfix(16)  OutScaling=2^0
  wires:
  Discrete Zero-Pole/1 -> Out1/1
  In1/1 -> Discrete Zero-Pole/1

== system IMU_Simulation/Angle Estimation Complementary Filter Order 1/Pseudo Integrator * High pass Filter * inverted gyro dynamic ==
  In1 : Inport  OutDataType=sfix(16)  OutScaling=2^0
  Discrete Zero-Pole : DiscreteZeroPole  Zeros=zerosd  Poles=polesd  Gain=gaind  SampleTime=SampleTime
  Out1 : Outport  OutDataType=sfix(16)  OutScaling=2^0
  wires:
  Discrete Zero-Pole/1 -> Out1/1
  In1/1 -> Discrete Zero-Pole/1

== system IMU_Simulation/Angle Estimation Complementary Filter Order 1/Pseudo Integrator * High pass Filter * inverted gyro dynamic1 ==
  In1 : Inport  OutDataType=sfix(16)  OutScaling=2^0
  Discrete Zero-Pole : DiscreteZeroPole  Zeros=zerosd  Poles=polesd  Gain=gaind  SampleTime=SampleTime
  Out1 : Outport  OutDataType=sfix(16)  OutScaling=2^0
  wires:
  In1/1 -> Discrete Zero-Pole/1
  Discrete Zero-Pole/1 -> Out1/1

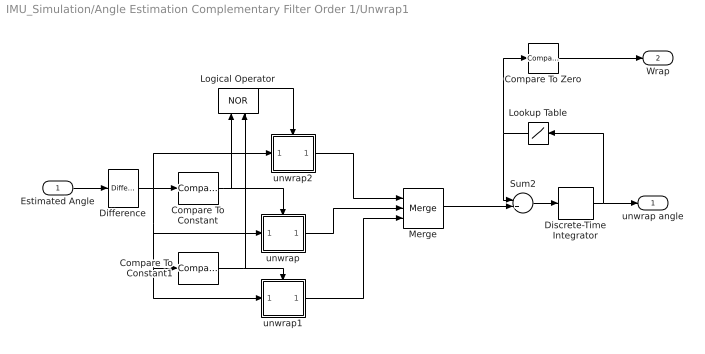
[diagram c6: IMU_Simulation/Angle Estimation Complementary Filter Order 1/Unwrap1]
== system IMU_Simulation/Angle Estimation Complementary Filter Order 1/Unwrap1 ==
  Estimated Angle : Inport
  Compare To Constant : simulink/Logic and Bit Operations/Compare To Constant  SystemSampleTime=-1  relop=>  const=180  LogicOutDataTypeMode=uint8  ZeroCross=off
  Compare To Constant1 : simulink/Logic and Bit Operations/Compare To Constant  SystemSampleTime=-1  relop=<  const=-180  LogicOutDataTypeMode=uint8  ZeroCross=off
  Compare To Zero : simulink/Logic and Bit Operations/Compare To Zero  SystemSampleTime=-1  relop=~=  LogicOutDataTypeMode=uint8  ZeroCross=off
  Difference : simulink/Discrete/Difference  SystemSampleTime=-1  ICPrevInput=0.0  OutDataType=sfix(16)  OutScaling=2^-10  DoSatur=off
  Discrete-Time Integrator : DiscreteIntegrator  gainval=1000  SampleTime=-1  OutDataType=sfix(16)  OutScaling=2^0  ICPrevOutput=DiscIntNeverNeededParam  ICPrevScaledInput=DiscIntNeverNeededParam
  Logical Operator : Logic  Orientation=up  Operator=NOR  AllPortsSameDT=off  OutDataTypeMode=boolean
  Lookup Table : Lookup  Orientation=left  InputValues=[-500 -195 195]  OutputValues=[+360 0 -360]  LookUpMeth=Use Input Below  OutDataType=sfix(16)  OutScaling=2^0
  Merge : Merge  Inputs=3
  Sum2 : Sum  OutDataType=sfix(16)  OutScaling=2^0
  unwrap : Subsystem  TreatAsAtomicUnit=on
  unwrap1 : Subsystem  TreatAsAtomicUnit=on
  unwrap2 : Subsystem  TreatAsAtomicUnit=on
  unwrap angle : Outport
  Wrap : Outport  Port=2
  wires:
  Discrete-Time Integrator/1 -> unwrap angle/1, Lookup Table/1
  Estimated Angle/1 -> Difference/1
  unwrap1/1(Out1) -> Merge/3
  unwrap/1(Out1) -> Merge/2
  unwrap2/1(Out1) -> Merge/1
  Logical Operator/1 -> unwrap2/Enable
  Compare To Constant1/1 -> Logical Operator/2, unwrap1/Enable
  Compare To Constant/1 -> unwrap/Enable, Logical Operator/1
  Difference/1 -> unwrap2/1(In1), unwrap1/1(In1), Compare To Constant1/1, unwrap/1(In1), Compare To Constant/1
  Sum2/1 -> Discrete-Time Integrator/1
  Merge/1 -> Sum2/2
  Lookup Table/1 -> Sum2/1, Compare To Zero/1
  Compare To Zero/1 -> Wrap/1

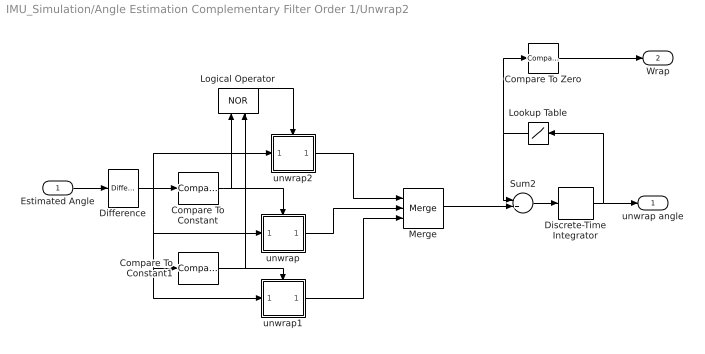
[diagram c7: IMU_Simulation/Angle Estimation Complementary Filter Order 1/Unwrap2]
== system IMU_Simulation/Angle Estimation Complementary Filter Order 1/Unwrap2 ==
  Estimated Angle : Inport
  Compare To Constant : simulink/Logic and Bit Operations/Compare To Constant  SystemSampleTime=-1  relop=>  const=180  LogicOutDataTypeMode=uint8  ZeroCross=off
  Compare To Constant1 : simulink/Logic and Bit Operations/Compare To Constant  SystemSampleTime=-1  relop=<  const=-180  LogicOutDataTypeMode=uint8  ZeroCross=off
  Compare To Zero : simulink/Logic and Bit Operations/Compare To Zero  SystemSampleTime=-1  relop=~=  LogicOutDataTypeMode=uint8  ZeroCross=off
  Difference : simulink/Discrete/Difference  SystemSampleTime=-1  ICPrevInput=0.0  OutDataType=sfix(16)  OutScaling=2^-10  DoSatur=off
  Discrete-Time Integrator : DiscreteIntegrator  gainval=1000  SampleTime=-1  OutDataType=sfix(16)  OutScaling=2^0  ICPrevOutput=DiscIntNeverNeededParam  ICPrevScaledInput=DiscIntNeverNeededParam
  Logical Operator : Logic  Orientation=up  Operator=NOR  AllPortsSameDT=off  OutDataTypeMode=boolean
  Lookup Table : Lookup  Orientation=left  InputValues=[-500 -195 195]  OutputValues=[+360 0 -360]  LookUpMeth=Use Input Below  OutDataType=sfix(16)  OutScaling=2^0
  Merge : Merge  Inputs=3
  Sum2 : Sum  OutDataType=sfix(16)  OutScaling=2^0
  unwrap : Subsystem  TreatAsAtomicUnit=on
  unwrap1 : Subsystem  TreatAsAtomicUnit=on
  unwrap2 : Subsystem  TreatAsAtomicUnit=on
  unwrap angle : Outport
  Wrap : Outport  Port=2
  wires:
  Compare To Zero/1 -> Wrap/1
  Lookup Table/1 -> Compare To Zero/1, Sum2/1
  Merge/1 -> Sum2/2
  Sum2/1 -> Discrete-Time Integrator/1
  Difference/1 -> Compare To Constant/1, unwrap/1(In1), Compare To Constant1/1, unwrap1/1(In1), unwrap2/1(In1)
  Compare To Constant/1 -> Logical Operator/1, unwrap/Enable
  Compare To Constant1/1 -> unwrap1/Enable, Logical Operator/2
  Logical Operator/1 -> unwrap2/Enable
  unwrap2/1(Out1) -> Merge/1
  unwrap/1(Out1) -> Merge/2
  unwrap1/1(Out1) -> Merge/3
  Estimated Angle/1 -> Difference/1
  Discrete-Time Integrator/1 -> Lookup Table/1, unwrap angle/1

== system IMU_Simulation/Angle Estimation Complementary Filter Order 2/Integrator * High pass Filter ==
  In1 : Inport  OutDataType=sfix(16)  OutScaling=2^0
  Discrete Zero-Pole : DiscreteZeroPole  Zeros=zerosd  Poles=polesd  Gain=gaind  SampleTime=SampleTime
  Out1 : Outport  OutDataType=sfix(16)  OutScaling=2^0
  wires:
  Discrete Zero-Pole/1 -> Out1/1
  In1/1 -> Discrete Zero-Pole/1

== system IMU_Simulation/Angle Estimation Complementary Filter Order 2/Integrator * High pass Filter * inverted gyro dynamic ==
  In1 : Inport  OutDataType=sfix(16)  OutScaling=2^0
  Discrete Zero-Pole : DiscreteZeroPole  Zeros=zerosd  Poles=polesd  Gain=gaind  SampleTime=SampleTime
  Out1 : Outport  OutDataType=sfix(16)  OutScaling=2^0
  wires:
  Discrete Zero-Pole/1 -> Out1/1
  In1/1 -> Discrete Zero-Pole/1

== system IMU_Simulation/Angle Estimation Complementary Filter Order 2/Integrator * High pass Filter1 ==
  In1 : Inport  OutDataType=sfix(16)  OutScaling=2^0
  Discrete Zero-Pole : DiscreteZeroPole  Zeros=zerosd  Poles=polesd  Gain=gaind  SampleTime=SampleTime
  Out1 : Outport  OutDataType=sfix(16)  OutScaling=2^0
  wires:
  In1/1 -> Discrete Zero-Pole/1
  Discrete Zero-Pole/1 -> Out1/1

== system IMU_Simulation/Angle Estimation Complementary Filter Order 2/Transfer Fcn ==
  In1 : Inport  OutDataType=sfix(16)  OutScaling=2^0
  Discrete Transfer Fcn : DiscreteTransferFcn  Numerator=numd  Denominator=dend  SampleTime=SampleTime
  Out1 : Outport  OutDataType=sfix(16)  OutScaling=2^0
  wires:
  In1/1 -> Discrete Transfer Fcn/1
  Discrete Transfer Fcn/1 -> Out1/1

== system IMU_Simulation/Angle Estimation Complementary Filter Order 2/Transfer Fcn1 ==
  In1 : Inport  OutDataType=sfix(16)  OutScaling=2^0
  Discrete Transfer Fcn : DiscreteTransferFcn  Numerator=numd  Denominator=dend  SampleTime=SampleTime
  Out1 : Outport  OutDataType=sfix(16)  OutScaling=2^0
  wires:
  Discrete Transfer Fcn/1 -> Out1/1
  In1/1 -> Discrete Transfer Fcn/1

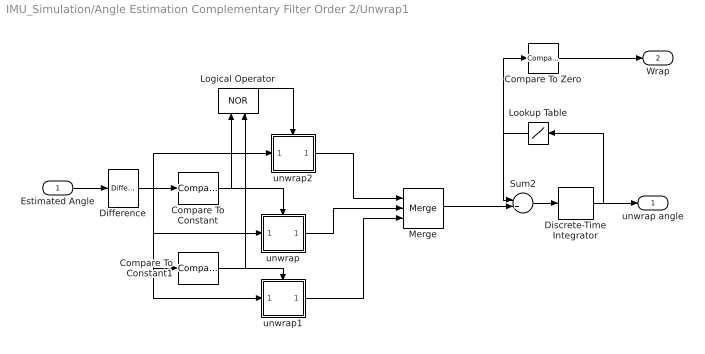
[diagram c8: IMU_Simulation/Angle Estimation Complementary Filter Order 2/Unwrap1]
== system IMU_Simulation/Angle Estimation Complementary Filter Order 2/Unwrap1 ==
  Estimated Angle : Inport
  Compare To Constant : simulink/Logic and Bit Operations/Compare To Constant  SystemSampleTime=-1  relop=>  const=180  LogicOutDataTypeMode=uint8  ZeroCross=off
  Compare To Constant1 : simulink/Logic and Bit Operations/Compare To Constant  SystemSampleTime=-1  relop=<  const=-180  LogicOutDataTypeMode=uint8  ZeroCross=off
  Compare To Zero : simulink/Logic and Bit Operations/Compare To Zero  SystemSampleTime=-1  relop=~=  LogicOutDataTypeMode=uint8  ZeroCross=off
  Difference : simulink/Discrete/Difference  SystemSampleTime=-1  ICPrevInput=0.0  OutDataType=sfix(16)  OutScaling=2^-10  DoSatur=off
  Discrete-Time Integrator : DiscreteIntegrator  gainval=1000  SampleTime=-1  OutDataType=sfix(16)  OutScaling=2^0  ICPrevOutput=DiscIntNeverNeededParam  ICPrevScaledInput=DiscIntNeverNeededParam
  Logical Operator : Logic  Orientation=up  Operator=NOR  AllPortsSameDT=off  OutDataTypeMode=boolean
  Lookup Table : Lookup  Orientation=left  InputValues=[-500 -195 195]  OutputValues=[+360 0 -360]  LookUpMeth=Use Input Below  OutDataType=sfix(16)  OutScaling=2^0
  Merge : Merge  Inputs=3
  Sum2 : Sum  OutDataType=sfix(16)  OutScaling=2^0
  unwrap : Subsystem  TreatAsAtomicUnit=on
  unwrap1 : Subsystem  TreatAsAtomicUnit=on
  unwrap2 : Subsystem  TreatAsAtomicUnit=on
  unwrap angle : Outport
  Wrap : Outport  Port=2
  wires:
  Compare To Zero/1 -> Wrap/1
  Lookup Table/1 -> Compare To Zero/1, Sum2/1
  Merge/1 -> Sum2/2
  Sum2/1 -> Discrete-Time Integrator/1
  Difference/1 -> Compare To Constant/1, unwrap/1(In1), Compare To Constant1/1, unwrap1/1(In1), unwrap2/1(In1)
  Compare To Constant/1 -> Logical Operator/1, unwrap/Enable
  Compare To Constant1/1 -> unwrap1/Enable, Logical Operator/2
  Logical Operator/1 -> unwrap2/Enable
  unwrap2/1(Out1) -> Merge/1
  unwrap/1(Out1) -> Merge/2
  unwrap1/1(Out1) -> Merge/3
  Estimated Angle/1 -> Difference/1
  Discrete-Time Integrator/1 -> Lookup Table/1, unwrap angle/1

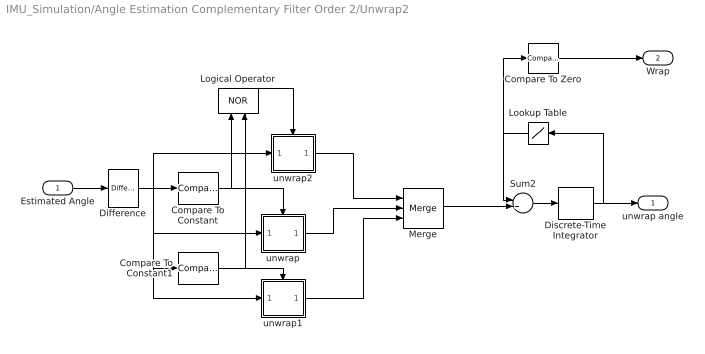
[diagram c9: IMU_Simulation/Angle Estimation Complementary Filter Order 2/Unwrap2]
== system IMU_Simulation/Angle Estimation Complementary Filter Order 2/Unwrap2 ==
  Estimated Angle : Inport
  Compare To Constant : simulink/Logic and Bit Operations/Compare To Constant  SystemSampleTime=-1  relop=>  const=180  LogicOutDataTypeMode=uint8  ZeroCross=off
  Compare To Constant1 : simulink/Logic and Bit Operations/Compare To Constant  SystemSampleTime=-1  relop=<  const=-180  LogicOutDataTypeMode=uint8  ZeroCross=off
  Compare To Zero : simulink/Logic and Bit Operations/Compare To Zero  SystemSampleTime=-1  relop=~=  LogicOutDataTypeMode=uint8  ZeroCross=off
  Difference : simulink/Discrete/Difference  SystemSampleTime=-1  ICPrevInput=0.0  OutDataType=sfix(16)  OutScaling=2^-10  DoSatur=off
  Discrete-Time Integrator : DiscreteIntegrator  gainval=1000  SampleTime=-1  OutDataType=sfix(16)  OutScaling=2^0  ICPrevOutput=DiscIntNeverNeededParam  ICPrevScaledInput=DiscIntNeverNeededParam
  Logical Operator : Logic  Orientation=up  Operator=NOR  AllPortsSameDT=off  OutDataTypeMode=boolean
  Lookup Table : Lookup  Orientation=left  InputValues=[-500 -195 195]  OutputValues=[+360 0 -360]  LookUpMeth=Use Input Below  OutDataType=sfix(16)  OutScaling=2^0
  Merge : Merge  Inputs=3
  Sum2 : Sum  OutDataType=sfix(16)  OutScaling=2^0
  unwrap : Subsystem  TreatAsAtomicUnit=on
  unwrap1 : Subsystem  TreatAsAtomicUnit=on
  unwrap2 : Subsystem  TreatAsAtomicUnit=on
  unwrap angle : Outport
  Wrap : Outport  Port=2
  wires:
  Discrete-Time Integrator/1 -> unwrap angle/1, Lookup Table/1
  Estimated Angle/1 -> Difference/1
  unwrap1/1(Out1) -> Merge/3
  unwrap/1(Out1) -> Merge/2
  unwrap2/1(Out1) -> Merge/1
  Logical Operator/1 -> unwrap2/Enable
  Compare To Constant1/1 -> Logical Operator/2, unwrap1/Enable
  Compare To Constant/1 -> unwrap/Enable, Logical Operator/1
  Difference/1 -> unwrap2/1(In1), unwrap1/1(In1), Compare To Constant1/1, unwrap/1(In1), Compare To Constant/1
  Sum2/1 -> Discrete-Time Integrator/1
  Merge/1 -> Sum2/2
  Lookup Table/1 -> Sum2/1, Compare To Zero/1
  Compare To Zero/1 -> Wrap/1

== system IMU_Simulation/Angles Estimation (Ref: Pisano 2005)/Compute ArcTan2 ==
  Force 1 : Inport
  Force 2 : Inport  Port=2
  Enable : EnablePort  StatesWhenEnabling=reset
  Gain1 : Gain  Gain=180/pi  ParameterDataType=sfix(16)  ParameterScaling=2^0  OutDataTypeMode=Specify via dialog  OutDataType=float('double')
  Trigonometric Function1 : Trigonometry  Operator=atan2  OutputSignalType=real
  Degree : Outport
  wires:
  Force 2/1 -> Trigonometric Function1/2
  Force 1/1 -> Trigonometric Function1/1
  Gain1/1 -> Degree/1
  Trigonometric Function1/1 -> Gain1/1

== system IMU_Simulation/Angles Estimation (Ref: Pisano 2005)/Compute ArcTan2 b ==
  Force 1 : Inport
  Force 2 : Inport  Port=2
  Enable : EnablePort  StatesWhenEnabling=reset
  Gain1 : Gain  Gain=180/pi  ParameterDataType=sfix(16)  ParameterScaling=2^0  OutDataTypeMode=Specify via dialog  OutDataType=float('double')
  Trigonometric Function1 : Trigonometry  Operator=atan2  OutputSignalType=real
  Degree : Outport
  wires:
  Trigonometric Function1/1 -> Gain1/1
  Gain1/1 -> Degree/1
  Force 1/1 -> Trigonometric Function1/1
  Force 2/1 -> Trigonometric Function1/2

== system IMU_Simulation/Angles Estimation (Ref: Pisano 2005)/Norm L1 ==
  Accel Y : Inport
  Accel Z : Inport  Port=2
  Accel X : Inport  Port=3
  Abs : Abs
  Abs1 : Abs
  Abs2 : Abs
  Sum1 : Sum  OutDataType=sfix(16)  OutScaling=2^0
  Sum3 : Sum  OutDataType=sfix(16)  OutScaling=2^0
  abs(Y)+abs(Z) : Outport
  abs(X)+abs(Z) : Outport  Port=2
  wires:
  Sum1/1 -> abs(X)+abs(Z)/1
  Accel X/1 -> Abs2/1
  Abs2/1 -> Sum1/2
  Sum3/1 -> abs(Y)+abs(Z)/1
  Accel Z/1 -> Abs1/1
  Accel Y/1 -> Abs/1
  Abs1/1 -> Sum3/2, Sum1/1
  Abs/1 -> Sum3/1

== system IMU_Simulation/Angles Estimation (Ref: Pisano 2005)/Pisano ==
  note: Probleme du filtrage de l'accelero : dephasage si variation rapide et de forte amplitude, fausse le calcul de l'offset Si on filtre moins, on se prend le biais du aux accelerations
  Gyro : Inport  Orientation=down
  Accel : Inport  Orientation=down  Port=2
  Adapt : Inport  Orientation=down  Port=3
  Constant : Constant  Orientation=left  Value=0  OutDataType=sfix(16)  OutScaling=2^0
  Gain6 : Gain  Orientation=left  Gain=1e-3  Multiplication=Matrix(K*u)  ParameterDataType=sfix(16)  ParameterScaling=2^0  OutDataType=sfix(16)  OutScaling=2^0
  Gain7 : Gain  Orientation=down  Gain=Ts  Multiplication=Matrix(K*u)  ParameterDataType=sfix(16)  ParameterScaling=2^0  OutDataType=sfix(16)  OutScaling=2^0
  Low Pass1 : Subsystem  Orientation=down  mask(DiscretizedZeroPole){Zeros=[], Poles=[-30*2*pi], Gain=30*2*pi, AbsTol=auto, SampleTime=.001, method=tustin, Wc=1}
      mask prompts: Zeros "Zeros (enter in s-main:)"; Poles "Poles (enter in s-domain:)"; Gain "Gain (enter in s-domain:)"; AbsTol "Absolute tolerance:"; SampleTime "Sample time:"; Wc "Critical Frequency (Hz):"
      mask help: Continuous mask uses c2d to transform parameters onto the Discrete Zero-Pole block inside.
      mask init:
      | st=SampleTime;
      | if length(st)>1
      |     st=SampleTime(1);
      | end
      | if(st>0)
      |     [zerosd,polesd,gaind] = sldiscutil('disczpk', {st,method,Wc,Zeros,Poles,Gain});
      | end	
      | s = get_param(gcb,'maskvalues');
      | zeross = s{1};
      | poless = s{2};
      | gainss = s{3};
      | %zerosc = eval(zeross);
      | %polesc = eval(poless);
      | %gainsc = eval(gainss);
      | sldiscutil('initzpkmask', st);
      | if(st==0)
      | set_param([gcb '/Zero Pole'], 'AbsoluteTolerance', AbsTol);
      | end
  Multiport Switch : MultiPortSwitch  Orientation=left  Inputs=2  zeroidx=on
  Sum2 : Sum  Inputs=++|  OutDataType=sfix(16)  OutScaling=2^0
  Sum4 : Sum  Inputs=++|  OutDataType=sfix(16)  OutScaling=2^0
  Sum5 : Sum  Orientation=left  Inputs=+-  OutDataType=sfix(16)  OutScaling=2^0
  Unit Delay2 : UnitDelay  SampleTime=-1
  Position : Outport  Orientation=up  OutDataType=sfix(16)  OutScaling=2^0
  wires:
  Low Pass1/1(Out1) -> Sum5/1
  Unit Delay2/1 -> Sum2/2, Sum5/2
  Gyro/1 -> Gain7/1
  Accel/1 -> Low Pass1/1(In1)
  Gain7/1 -> Sum2/1
  Sum5/1 -> Gain6/1
  Sum2/1 -> Sum4/2
  Multiport Switch/1 -> Sum4/1
  Adapt/1 -> Multiport Switch/1
  Gain6/1 -> Multiport Switch/3
  Constant/1 -> Multiport Switch/2
  Sum4/1 -> Position/1, Unit Delay2/1
